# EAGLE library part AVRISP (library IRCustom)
AVR ISP HEADER Standard 6 pin header for AVR programming
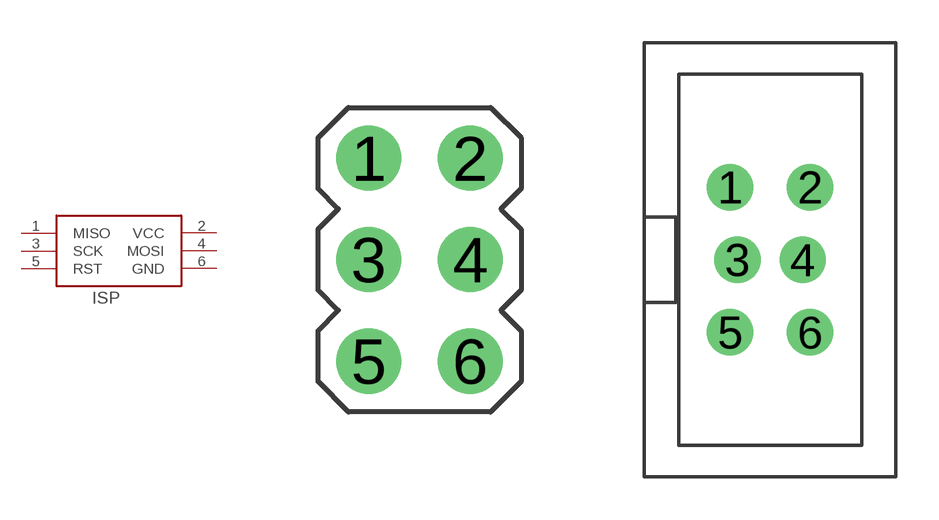
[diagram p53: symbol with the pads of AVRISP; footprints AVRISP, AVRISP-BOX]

Designator prefix ISP

## AVRISP-6  [AVRISP]
1  MISO  in
2  VCC  pwr
3  SCK  out
4  MOSI  out
5  RST  out
6  GND  pwr

## AVRISP-BOX  [AVRISP-BOX]
Pads as for AVRISP

## Footprint AVRISP (pad centres in mm)
drill 0.9 pad 1.626: 1 -1.27,2.54; 2 1.27,2.54; 3 -1.27,0; 4 1.27,0; 5 -1.27,-2.54; 6 1.27,-2.54

## Footprint AVRISP-BOX (pad centres in mm)
drill 0.9 pad 1.626: 1 -1.397,2.54; 2 1.397,2.54; 3 -1.143,0; 4 1.143,0; 5 -1.397,-2.54; 6 1.397,-2.54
